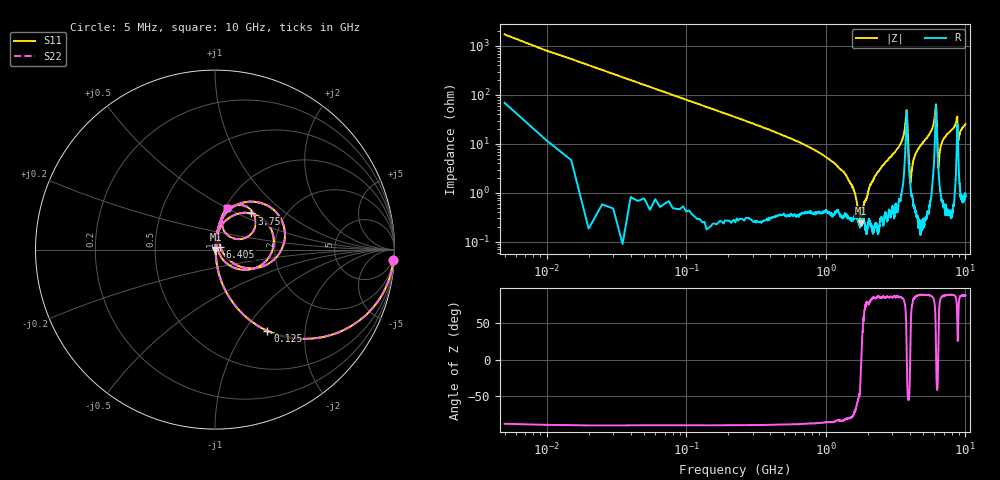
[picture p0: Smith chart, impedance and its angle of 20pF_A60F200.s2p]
! Amotech Co.,Ltd.
! http://www.amotech.co.kr/
! Part Number: A60F200
! These Parameters are Measured in Series Mode Connection
! Operation Temp=25[degC], DC Bias Voltage=0[V]
! Freq. Start=5[MHz] Stop=10[GHz], 2000[Steps]
! Date: Monday, July 20, 2020, 03:36:55
# GHZ S RI R 50.000000
!Freq.(Hz) S11(Real) S11(Imag) S21(Real) S21(Imag) S12(Real) S12(Imag) S22(Real) S22(Imag)
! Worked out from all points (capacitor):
!   2000 points, 5 MHz to 10 GHz, reference 50 ohm
!   read as one part in series: C = 19.8 pF near 55 MHz
!   lowest |Z| = 240 mohm at 1.795 GHz (marker M1)
!   series resonance near 1.797 GHz, so ESL is about 400 pH
!   S11 on the Smith chart (normalised r, x): 5 MHz: 2, -34; 125 MHz: 1.01, -1.28; 3.75 GHz: 1.36, +0.60; 6.405 GHz: 1.06, +0.03; 10 GHz: 1.02, +0.50
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0.005  0.9943 -0.0577  0.00568 0.0577  0.00568 0.0577  0.9943 -0.0577
0.065  0.6034 -0.4871  0.3966 0.4871  0.3966 0.4871  0.6034 -0.4871
0.125  0.2921 -0.4524  0.7079 0.4524  0.7079 0.4524  0.2921 -0.4524
0.365  0.0453 -0.2016  0.9547 0.2016  0.9547 0.2016  0.0453 -0.2016
1.38  0.00399 -0.0236  0.996 0.0236  0.996 0.0236  0.00399 -0.0236
1.675  0.00312 -0.00515  0.9969 0.00515  0.9969 0.00515  0.00312 -0.00515
1.795  0.00239 -8.77e-05  0.9976 8.77e-05  0.9976 8.77e-05  0.00239 -8.77e-05
2.26  0.00272 0.022  0.9973 -0.022  0.9973 -0.022  0.00272 0.022
3.34  0.0149 0.0855  0.9851 -0.0855  0.9851 -0.0855  0.0149 0.0855
3.75  0.2031 0.2015  0.7969 -0.2015  0.7969 -0.2015  0.2031 0.2015
3.825  0.2474 -0.0925  0.7526 0.0925  0.7526 0.0925  0.2474 -0.0925
4.045  0.0134 0.00803  0.9866 -0.00803  0.9866 -0.00803  0.0134 0.00803
4.36  0.00784 0.0579  0.9922 -0.0579  0.9922 -0.0579  0.00784 0.0579
5.005  0.0146 0.1086  0.9854 -0.1086  0.9854 -0.1086  0.0146 0.1086
5.885  0.0728 0.216  0.9272 -0.216  0.9272 -0.216  0.0728 0.216
6.135  0.3748 0.1554  0.6252 -0.1554  0.6252 -0.1554  0.3748 0.1554
6.405  0.0292 0.0134  0.9708 -0.0134  0.9708 -0.0134  0.0292 0.0134
6.67  0.0171 0.0878  0.9829 -0.0878  0.9829 -0.0878  0.0171 0.0878
8.335  0.0557 0.2126  0.9443 -0.2126  0.9443 -0.2126  0.0557 0.2126
8.72  0.2006 0.2198  0.7994 -0.2198  0.7994 -0.2198  0.2006 0.2198
8.9  0.0637 0.0873  0.9363 -0.0873  0.9363 -0.0873  0.0637 0.0873
10  0.0677 0.2332  0.9323 -0.2332  0.9323 -0.2332  0.0677 0.2332
